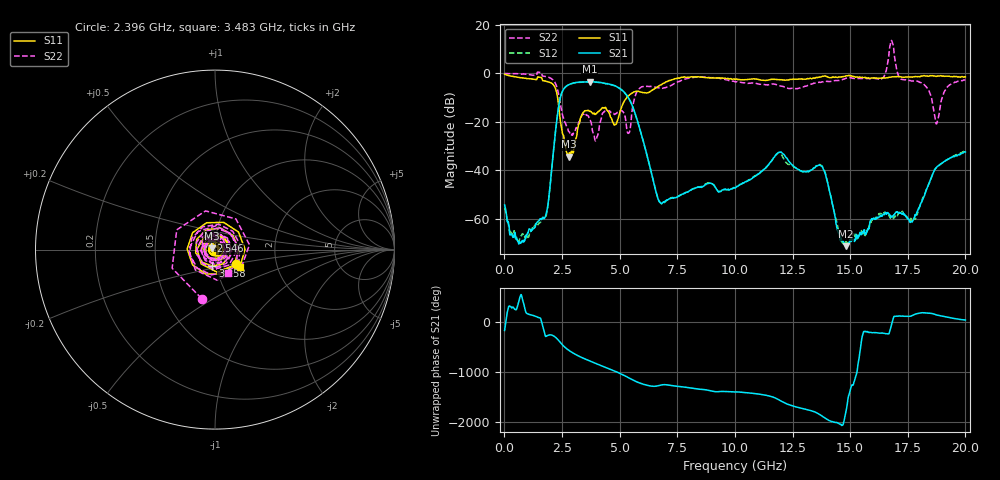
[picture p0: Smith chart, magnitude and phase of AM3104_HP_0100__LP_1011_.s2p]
!Created with skrf (http://scikit-rf.org).
# Hz S RI R 50.0
!freq ReS11 ImS11 ReS21 ImS21 ReS12 ImS12 ReS22 ImS22
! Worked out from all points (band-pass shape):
!   1601 points, 10 MHz to 20 GHz, reference 50 ohm
!   highest |S21| = -3.43 dB at 3.696 GHz (marker M1); lowest = -71.4 dB at 14.82 GHz (marker M2)
!   |S21| within 3 dB of the highest: 2.574 GHz to 5.037 GHz (2.464 GHz wide, 64.7 % of centre)
!   lowest |S11| = -34.3 dB at 2.796 GHz (marker M3), VSWR 1.04, Z = 48.2 + j0.676 ohm
!   |S11| at or under -10 dB: 2.308 GHz to 5.305 GHz (2.996 GHz wide, 78.7 % of centre)
!   |S22| runs from -27.9 to 13.6 dB; largest |S21 - S12| = 0.055
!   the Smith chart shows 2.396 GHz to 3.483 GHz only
!   S11 on the Smith chart (normalised r, x): 2.396 GHz: 1.25, -0.21; 2.546 GHz: 0.95, +0.09; 3.258 GHz: 0.95, -0.18; 3.483 GHz: 1.29, -0.25
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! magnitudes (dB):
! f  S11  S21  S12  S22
! 10 MHz  -0.3  -54.3  -55.6  0.0
! 659.7 MHz  -1.7  -69.9  -68.4  -0.2
! 1.747 GHz  -3.1  -59.7  -59.7  -1.2
! 2.396 GHz  -16.8  -11.4  -11.5  -11.0
! 2.546 GHz  -25.4  -6.8  -6.9  -17.9
! 2.796 GHz  -34.3  -4.6  -4.6  -24.0
! 3.258 GHz  -20.6  -3.6  -3.7  -19.8
! 3.346 GHz  -17.6  -3.6  -3.6  -17.5
! 3.483 GHz  -15.5  -3.5  -3.6  -16.5
! 3.696 GHz  -15.6  -3.4  -3.5  -19.2
! 5.382 GHz  -9.3  -10.1  -10.1  -24.7
! 5.807 GHz  -7.4  -20.7  -20.7  -6.8
! 6.682 GHz  -5.3  -52.2  -52.0  -5.9
! 10.01 GHz  -2.5  -47.4  -47.3  -3.4
! 11.93 GHz  -2.5  -32.5  -32.8  -5.1
! 13.34 GHz  -2.1  -39.8  -39.8  -4.4
! 13.85 GHz  -1.1  -39.8  -39.4  -3.4
! 14.82 GHz  -1.0  -71.4  -69.8  -2.0
! 16.68 GHz  -1.6  -58.0  -58.7  7.2
! 17.69 GHz  -1.5  -61.4  -60.4  -3.1
! 18.75 GHz  -1.2  -38.8  -38.8  -20.9
! 20 GHz  -1.4  -32.5  -31.8  -2.6
